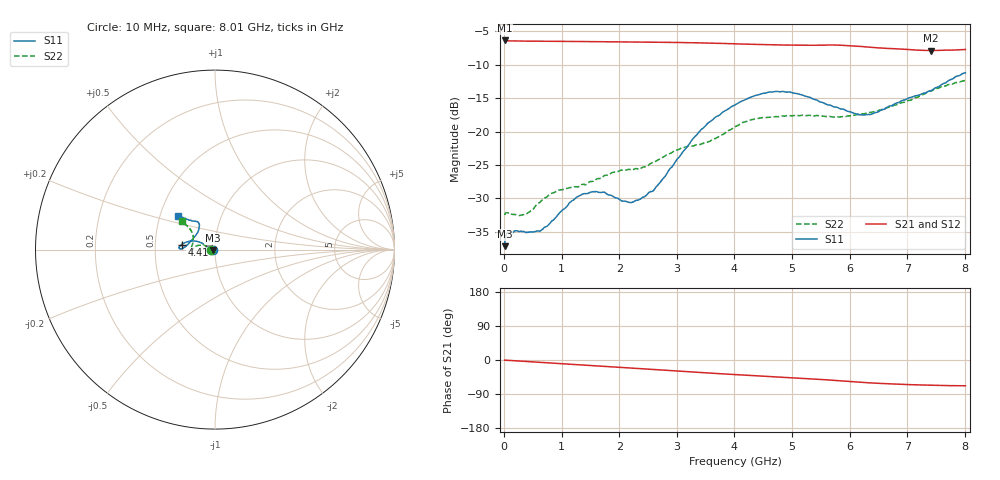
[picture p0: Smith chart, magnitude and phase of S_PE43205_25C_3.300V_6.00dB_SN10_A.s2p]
! Device ID: PE43205
! Dir: z:\David_A\43205\PE43701\25C\3p300V\0p25dB
! Serial: 10
! Insertion: A
! Impedance: 50 ohm
! Temp: 25C
! VDD: 3.300V
! Attenuation Step: 0.25dB
! IDD: 1.234558e-01mA
#  Hz  S  RI  R  50
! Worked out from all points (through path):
!   801 points, 10 MHz to 8.01 GHz, reference 50 ohm
!   highest |S21| = -6.35 dB at 10 MHz (marker M1); lowest = -7.9 dB at 7.41 GHz (marker M2)
!   group delay of S21, straight-line fit = 25 ps
!   lowest |S11| = -37.2 dB at 10 MHz (marker M3), VSWR 1.03, Z = 48.7 - j0.402 ohm
!   |S11| at or under -10 dB: start of sweep to end of sweep
!   |S22| runs from -32.6 to -12.3 dB; largest |S21 - S12| = 0.0023
!   S11 on the Smith chart (normalised r, x): 10 MHz: 0.97, -0.01; 4.41 GHz: 0.69, +0.04; 8.01 GHz: 0.62, +0.25
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1e7  -0.0133 -0.00413  0.4816 -0.00314  0.4812 -0.00327  -0.0237 -0.000979
9e7  -0.0175 -0.00116  0.4782 -0.00879  0.4782 -0.00883  -0.0245 0.00173
3.6e8  -0.0176 -0.00256  0.4765 -0.0312  0.4763 -0.0307  -0.0229 0.00705
6.4e8  -0.0171 -0.00619  0.4724 -0.053  0.4725 -0.0532  -0.0282 0.0104
9.3e8  -0.0203 -0.0121  0.468 -0.0755  0.4681 -0.0756  -0.0354 0.00728
1.35e9  -0.0262 -0.0215  0.4597 -0.1078  0.4597 -0.1079  -0.0401 0.00297
1.72e9  -0.025 -0.0248  0.451 -0.1353  0.4509 -0.1355  -0.0458 0.00527
2.21e9  -0.0273 -0.0109  0.437 -0.1705  0.4369 -0.1705  -0.0508 0.0105
2.43e9  -0.0324 -0.00241  0.4297 -0.1861  0.4296 -0.186  -0.0518 0.0168
2.68e9  -0.0392 0.0096  0.4206 -0.2036  0.4204 -0.2036  -0.0568 0.0243
3.09e9  -0.0623 0.0298  0.4028 -0.2308  0.4029 -0.2309  -0.0705 0.028
3.41e9  -0.0922 0.0439  0.3879 -0.2506  0.3878 -0.2508  -0.0764 0.0242
4.01e9  -0.1525 0.0439  0.3549 -0.2837  0.3548 -0.2837  -0.1071 0.0185
4.41e9  -0.1863 0.0273  0.3339 -0.3009  0.334 -0.3009  -0.1256 -0.00159
4.85e9  -0.1996 0.00927  0.3109 -0.3186  0.3108 -0.3183  -0.1307 -0.00876
5.35e9  -0.1766 0.00844  0.2849 -0.3397  0.2849 -0.3394  -0.131 0.00847
5.81e9  -0.1462 0.0348  0.2572 -0.3623  0.2569 -0.3625  -0.124 0.0344
6.2e9  -0.1118 0.0728  0.2245 -0.3718  0.2252 -0.3717  -0.1212 0.0595
6.39e9  -0.0977 0.0949  0.2094 -0.3728  0.2094 -0.3726  -0.1204 0.0714
6.68e9  -0.089 0.1268  0.1916 -0.3732  0.1919 -0.3725  -0.126 0.0858
7.41e9  -0.1256 0.1589  0.1616 -0.3713  0.1617 -0.3716  -0.1542 0.1299
8.01e9  -0.2046 0.1848  0.1542 -0.3822  0.153 -0.3842  -0.1839 0.1574
